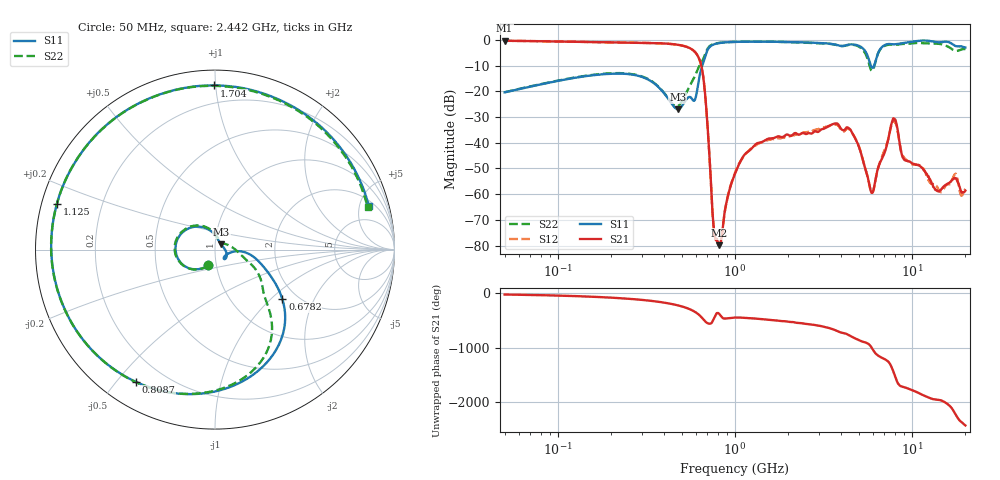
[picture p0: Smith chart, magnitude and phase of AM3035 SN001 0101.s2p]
# Hz S DB R 50
!freq MagS11 AngS11 MagS21 AngS21 MagS12 AngS12 MagS22 AngS22
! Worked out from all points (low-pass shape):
!   1601 points, 50 MHz to 20.05 GHz, reference 50 ohm
!   highest |S21| = -0.38 dB at 50 MHz (marker M1); lowest = -79.8 dB at 814.8 MHz (marker M2)
!   |S21| within 3 dB of the highest: start of sweep to 561 MHz
!   lowest |S11| = -27.0 dB at 475.1 MHz (marker M3), VSWR 1.09, Z = 53.5 + j3.08 ohm
!   |S11| at or under -10 dB: start of sweep to 654.8 MHz; 5.86 GHz to 6.121 GHz (260.6 MHz wide, 4.35 % of centre)
!   |S22| runs from -25.9 to -0.7 dB; largest |S21 - S12| = 0.0041
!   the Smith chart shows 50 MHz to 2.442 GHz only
!   S11 on the Smith chart (normalised r, x): 50 MHz: 0.92, -0.16; 678.2 MHz: 1.68, -1.18; 808.7 MHz: 0.10, -0.56; 1.125 GHz: 0.04, +0.14; 1.704 GHz: 0.09, +0.99; 2.442 GHz: 2.65, +6.17
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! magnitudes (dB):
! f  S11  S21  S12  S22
! 50 MHz  -20.4  -0.4  -0.4  -20.4
! 135.9 MHz  -14.4  -0.8  -0.8  -14.2
! 369.6 MHz  -18.3  -1.3  -1.3  -18.2
! 475.1 MHz  -27.0  -1.9  -1.9  -25.8
! 615.2 MHz  -18.6  -6.1  -6.1  -11.7
! 678.2 MHz  -6.6  -20.9  -20.9  -5.7
! 758.8 MHz  -1.8  -72.9  -72.9  -1.6
! 808.7 MHz  -1.3  -79.5  -79.7  -1.2
! 814.8 MHz  -1.3  -79.8  -80.1  -1.2
! 1.005 GHz  -0.8  -51.8  -51.3  -0.8
! 1.125 GHz  -0.8  -44.9  -45.2  -0.7
! 1.704 GHz  -0.8  -37.8  -38.2  -0.8
! 2.442 GHz  -1.0  -36.3  -36.0  -1.1
! 2.722 GHz  -1.1  -36.4  -35.5  -1.2
! 4.43 GHz  -1.9  -34.5  -34.8  -1.9
! 5.956 GHz  -10.8  -59.4  -59.5  -12.1
! 7.402 GHz  -1.6  -37.6  -37.7  -1.9
! 7.978 GHz  -1.8  -30.8  -31.7  -2.0
! 9.095 GHz  -1.2  -46.8  -46.1  -1.6
! 14.42 GHz  -1.0  -58.5  -59.0  -1.6
! 17.52 GHz  -2.3  -53.8  -52.2  -4.2
! 20.05 GHz  -3.0  -58.6  -58.0  -3.6
